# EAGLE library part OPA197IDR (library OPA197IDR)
36-V, Precision, Rail-to-Rail Input Output, Low Offset Voltage Op Amp Source: Datasheet
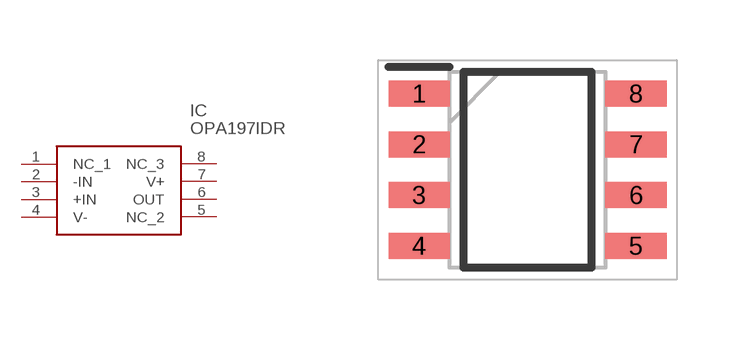
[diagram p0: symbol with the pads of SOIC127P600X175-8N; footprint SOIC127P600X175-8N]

Designator prefix IC

## OPA197IDR (Arrow_Part_Number: OPA197IDR; Arrow_Price-Stock: https://www.arrow.com/en/products/opa197idr/texas-instruments?utm_currency=USD&region=europe; Description: 36-V, Precision, Rail-to-Rail Input Output, Low Offset Voltage Op Amp; Height: 1.75mm; Manufacturer_Name: Texas Instruments; Manufacturer_Part_Number: OPA197IDR; Mouser_Part_Number: 595-OPA197IDR; Mouser_Price-Stock: https://www.mouser.co.uk/ProductDetail/Texas-Instruments/OPA197IDR?qs=gMfM3zrbS4ovW9KDi3YhFw%3D%3D)  [SOIC127P600X175-8N]
1  NC_1
2  -IN
3  +IN
4  V-
5  NC_2
6  OUT
7  V+
8  NC_3

## Footprint SOIC127P600X175-8N (pad centres in mm)
SOIC (8)(Height=1.75mm)
smd 1.528 x 0.65: 1 -2.711,1.905; 2 -2.711,0.635; 3 -2.711,-0.635; 4 -2.711,-1.905; 5 2.711,-1.905; 6 2.711,-0.635; 7 2.711,0.635; 8 2.711,1.905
